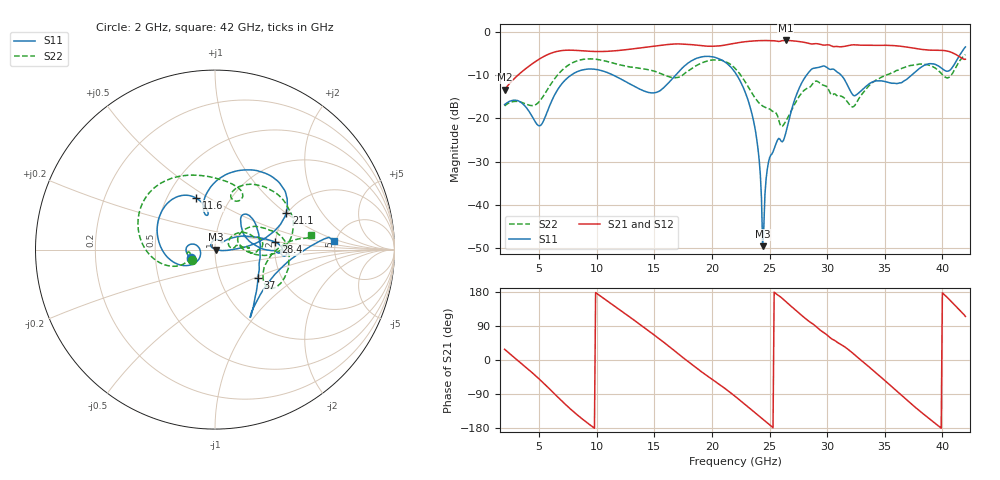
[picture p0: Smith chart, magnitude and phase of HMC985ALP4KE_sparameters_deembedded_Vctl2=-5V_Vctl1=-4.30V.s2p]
!s2p File: Measurements: S11, S21, S12, S22
# GHz S dB R 50.0
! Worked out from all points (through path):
!   401 points, 2 GHz to 42 GHz, reference 50 ohm
!   highest |S21| = -2.07 dB at 26.4 GHz (marker M1); lowest = -13.4 dB at 2 GHz (marker M2)
!   lowest |S11| = -49.5 dB at 24.4 GHz (marker M3), VSWR 1.01, Z = 50.3 + j0.0466 ohm
!   |S11| at or under -10 dB: start of sweep to 7.805 GHz; 22.14 GHz to 28.23 GHz (6.087 GHz wide, 24.2 % of centre); 31.19 GHz to 37.36 GHz (6.174 GHz wide, 18 % of centre)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
!   |S22| runs from -21.9 to -5.3 dB; largest |S21 - S12| = 0.00081
!   S11 on the Smith chart (normalised r, x): 2 GHz: 0.76, -0.07; 11.6 GHz: 0.69, +0.44; 21.1 GHz: 1.97, +1.01; 28.4 GHz: 2.00, +0.19; 37 GHz: 1.52, -0.53; 42 GHz: 4.79, +0.82
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2  -16.85 -161.8  -13.44 28.2  -13.44 28.2  -17.16 -155.7
5  -21.74 -172.7  -6.38 -50.1  -6.38 -50.1  -16.18 -159.9
6.3  -14.83 -150.5  -4.76 -88.3  -4.76 -88.3  -11.04 -161.6
8.7  -8.90 150.3  -4.44 -154.6  -4.44 -154.6  -6.48 151.3
11.6  -10.28 110.2  -4.45 141.0  -4.45 141.0  -7.41 103.5
13.6  -13.11 101.1  -3.85 97.1  -3.85 97.2  -8.45 75.9
15.4  -13.80 105.7  -3.25 56.4  -3.25 56.4  -9.54 62.4
17.9  -7.32 80.1  -2.95 -3.6  -2.94 -3.6  -9.15 72.3
21.1  -6.99 27.4  -3.14 -74.5  -3.14 -74.4  -6.88 16.1
22  -9.41 16.8  -2.71 -95.7  -2.71 -95.7  -8.48 0.7
23.6  -20.49 -0.2  -2.18 -135.4  -2.18 -135.4  -14.75 -3.8
24  -27.16 -7.3  -2.11 -145.4  -2.11 -145.4  -16.22 1.8
24.4  -49.50 7.9  -2.09 -155.5  -2.08 -155.5  -17.18 7.5
25  -29.12 133.3  -2.11 -170.8  -2.11 -170.8  -17.87 11.0
26.4  -23.48 42.9  -2.06 154.5  -2.06 154.5  -20.74 33.1
28.4  -9.41 7.1  -2.74 102.5  -2.74 102.5  -12.93 18.4
28.7  -8.60 2.1  -2.87 96.3  -2.88 96.4  -12.20 16.6
32.5  -14.67 33.4  -3.08 10.6  -3.08 10.6  -16.64 28.8
35.4  -11.77 18.9  -3.20 -64.9  -3.20 -64.8  -9.79 19.4
37  -10.83 -33.5  -3.62 -107.9  -3.62 -107.9  -8.02 5.1
39.8  -8.19 -56.8  -4.33 -177.4  -4.33 -177.4  -9.38 -34.9
42  -3.57 4.2  -6.40 115.0  -6.41 115.1  -5.31 8.8
